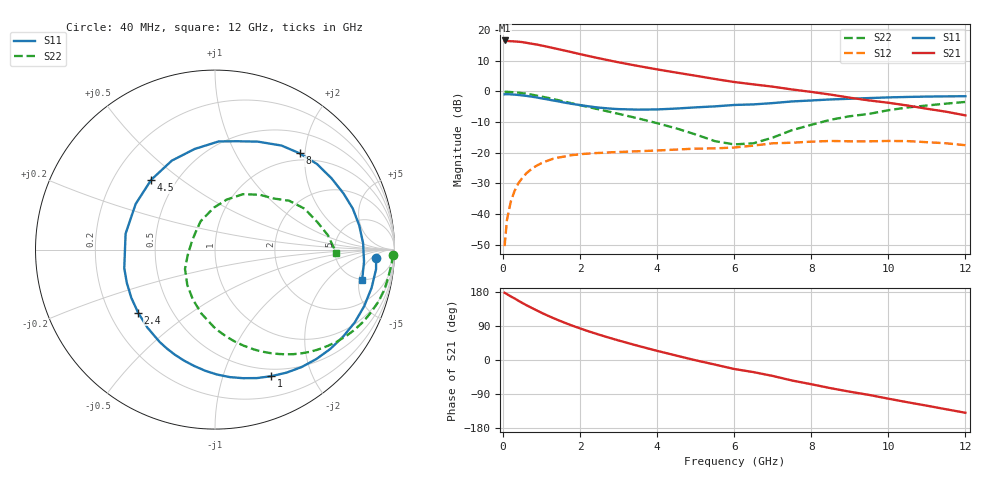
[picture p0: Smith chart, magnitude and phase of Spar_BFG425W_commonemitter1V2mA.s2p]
! Filename: 12bfg425.001
! BFG425W Field C1
! V1=8.096E-001V,V2=1.000E+000V, I1=2.742E-005A, I2=2.000E-003A
# GHz  S  MA  R 50
!  S11  S21  S12  S22
!Freq(GHz)  Mag  Ang  Mag  Ang  Mag  Ang  Mag  Ang
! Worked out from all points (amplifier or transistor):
!   44 points, 40 MHz to 12 GHz, reference 50 ohm
!   highest |S21| = 16.6 dB at 40 MHz (marker M1)
!   |S21| within 3 dB of that: start of sweep to 1.492 GHz
!   unconditionally stable (mu >= 1): 3.097 GHz to end of sweep
!   at 700 MHz: K = 0.19, MSG = 20.7 dB, |S12| = -25.7 dB
!   at 2.4 GHz: K = 0.73, MSG = 15.6 dB, |S12| = -20.1 dB
!   at 12 GHz: K = 1.77, MAG = -0.2 dB, |S12| = -17.5 dB
!   S11 on the Smith chart (normalised r, x): 40 MHz: 15, -7; 1 GHz: 0.42, -1.46; 2.4 GHz: 0.32, -0.32; 4.5 GHz: 0.36, +0.39; 8 GHz: 0.86, +1.89; 12 GHz: 4.95, -5.54
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0.04  0.899 -2.9  6.799 177.3  0.003 77.3  0.99 -1.7
0.1  0.904 -7.0  6.673 174.0  0.008 85.4  0.988 -4.3
0.2  0.898 -13.8  6.605 167.8  0.016 80.6  0.978 -9.0
0.3  0.889 -20.8  6.557 162.4  0.024 76.0  0.97 -13.2
0.5  0.863 -34.1  6.387 150.5  0.039 67.0  0.938 -21.6
0.6  0.848 -40.7  6.237 145.0  0.046 62.8  0.92 -25.7
0.8  0.813 -53.6  5.933 134.6  0.058 54.6  0.875 -33.4
1  0.772 -66.0  5.621 124.5  0.068 47.3  0.826 -40.5
1.3  0.715 -83.4  5.116 110.8  0.08 37.6  0.753 -50.1
1.6  0.658 -100.3  4.651 98.3  0.087 29.3  0.682 -58.5
1.9  0.613 -115.9  4.208 86.9  0.093 22.4  0.618 -66.2
2.2  0.575 -130.9  3.814 76.4  0.097 16.5  0.56 -73.2
2.4  0.554 -140.7  3.582 69.8  0.099 13.1  0.525 -77.7
3  0.516 -168.4  2.992 51.5  0.103 4.6  0.432 -90.8
3.5  0.506 169.9  2.61 37.4  0.106 -1.0  0.365 -101.9
4.5  0.527 132.4  2.032 11.6  0.113 -10.7  0.25 -128.2
5.5  0.572 101.4  1.599 -12.1  0.118 -20.6  0.155 -168.7
6.5  0.616 78.5  1.306 -32.0  0.131 -25.6  0.143 140.5
8  0.714 48.7  0.985 -63.9  0.152 -48.1  0.286 76.9
8.5  0.742 40.0  0.89 -74.3  0.156 -56.5  0.346 63.1
10.5  0.815 9.5  0.59 -111.5  0.155 -88.6  0.549 24.5
12  0.837 -11.5  0.408 -139.3  0.133 -118.0  0.675 -1.4
